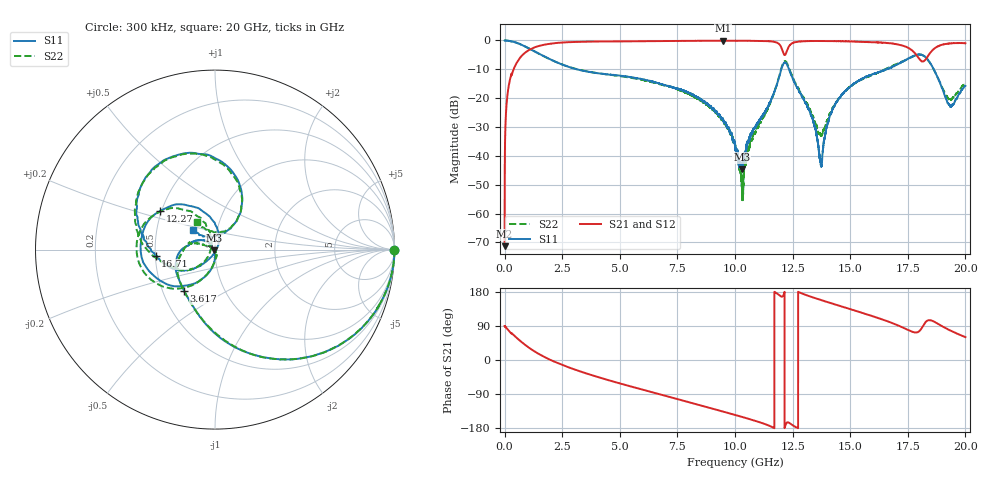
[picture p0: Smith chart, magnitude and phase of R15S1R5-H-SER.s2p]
!{R15S1R5}
!Johanson Technology Inc.
!www.johansontechnology.com
!Test Board Conditions:
!Substrate Type  RO4350B
!Substrate Thickness  20 mil
!Substrate Dk  3.66
!TL Type: GCPW
!TL Trace Width  34 mil
!TL Gap  10 mil
!Electrode orientation  Horizontal
!DUT TOPOLOGY	SERIES
!Mounting Pad LxW  26x52 mil
! Created Sat Feb  6 12:15:40 2021
# hz S ma R 50
! 2 Port Network Data from SP1.SP block
! freq  magS11  angS11  magS21  angS21  magS12  angS12  magS22  angS22
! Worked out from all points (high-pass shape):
!   20001 points, 300 kHz to 20 GHz, reference 50 ohm
!   highest |S21| = -0.08 dB at 9.474 GHz (marker M1); lowest = -71.3 dB at 300 kHz (marker M2)
!   |S21| within 3 dB of the highest: 1.111 GHz to 12.05 GHz (10.93 GHz wide, 166 % of centre); 12.28 GHz to 17.62 GHz (5.34 GHz wide, 35.7 % of centre)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
!   lowest |S11| = -44.6 dB at 10.29 GHz (marker M3), VSWR 1.01, Z = 49.6 - j0.445 ohm
!   |S11| at or under -10 dB: 3.143 GHz to 12.01 GHz (8.868 GHz wide, 117 % of centre); 12.35 GHz to 16.58 GHz (4.237 GHz wide, 29.3 % of centre); 18.63 GHz to end of sweep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
!   |S22| runs from -56.0 to 0.0 dB; largest |S21 - S12| = 0.017
!   S11 on the Smith chart (normalised r, x): 300 kHz: open; 3.617 GHz: 0.64, -0.32; 12.27 GHz: 0.49, +0.25; 16.71 GHz: 0.50, -0.04; 20 GHz: 0.77, +0.18
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300000  0.9951 -0.1  0.000272 89.1  0.0002784 92.4  0.9951 -0.1
1.343e8  0.9916 -9.0  0.1231 80.7  0.1237 80.8  0.9917 -8.9
5.073e8  0.916 -30.2  0.3978 59.4  0.3988 59.5  0.9143 -30.3
1.7313e9  0.5267 -82.1  0.8444 8.0  0.8463 8.0  0.5256 -81.6
3.3343e9  0.303 -121.0  0.9478 -31.2  0.9485 -31.1  0.3047 -120.6
3.6173e9  0.288 -126.6  0.9529 -36.8  0.953 -36.8  0.2889 -126.2
6.6673e9  0.1818 178.9  0.9751 -89.4  0.9753 -89.4  0.1772 -178.6
9.4743e9  0.04222 132.3  0.9906 -136.0  0.9902 -136.1  0.04341 150.5
1.00003e10  0.0155 144.9  0.9892 -145.0  0.9897 -144.9  0.01618 145.9
1.02893e10  0.005876 -130.3  0.9878 -149.9  0.9872 -149.9  0.003678 -146.4
1.19633e10  0.2699 -131.3  0.8203 169.1  0.822 169.2  0.2795 -130.0
1.22663e10  0.3734 144.6  0.6842 -164.5  0.6817 -165.0  0.3963 151.9
1.33343e10  0.0473 61.8  0.977 166.2  0.9763 166.3  0.05135 111.7
1.37313e10  0.007372 -29.6  0.9788 158.4  0.9774 158.4  0.02237 170.5
1.40663e10  0.04188 -114.8  0.9765 152.0  0.9789 151.9  0.04717 -139.4
1.45793e10  0.1055 -131.0  0.974 142.1  0.9711 142.2  0.1073 -132.5
1.66673e10  0.3248 -173.4  0.9002 101.0  0.8847 100.9  0.3378 -172.8
1.67063e10  0.3326 -174.0  0.8938 100.2  0.8868 100.1  0.3461 -173.9
1.81403e10  0.5563 104.2  0.4337 88.0  0.43 88.4  0.5557 106.1
1.85653e10  0.3518 65.1  0.6734 103.4  0.6723 103.6  0.3466 65.6
1.93123e10  0.07515 89.0  0.885 78.9  0.8852 79.0  0.09707 81.8
2e10  0.1633 137.1  0.8951 60.3  0.891 60.3  0.1852 122.6
